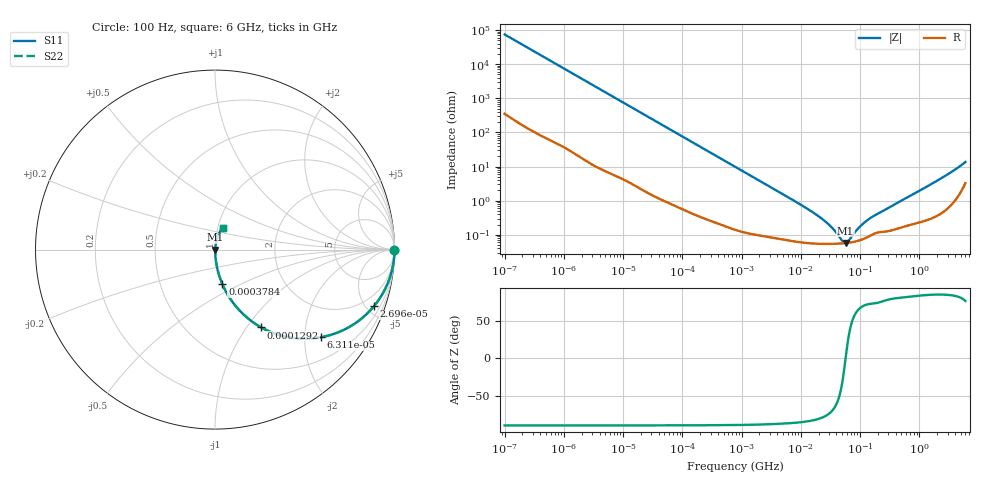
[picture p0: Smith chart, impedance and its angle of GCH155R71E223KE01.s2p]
!Murata Part Number: GCH155R71E223KE01
!These Parameters are Measured in Series Mode Connection
!Data Generated on Mar 13, 2026
!  o--ll--o
!Port1  Port2
!  o------o
!Operation Temp=25[degC], DC Bias Voltage=0[V]
!Freq. Start=100[Hz] Stop=6[GHz] 401[Steps]
# Hz S RI R 50
!Freq.(Hz) S11(Real) S11(Imag) S21(Real) S21(Imag) S12(Real) S12(Imag) S22(Real) S22(Imag)
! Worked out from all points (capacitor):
!   401 points, 100 Hz to 6 GHz, reference 50 ohm
!   read as one part in series: C = 21.5 nF near 109 Hz
!   lowest |Z| = 57.3 mohm at 56.99 MHz (marker M1)
!   series resonance near 57.05 MHz, so ESL is about 360 pH
!   S11 on the Smith chart (normalised r, x): 100 Hz: open; 26.96 kHz: 1.03, -5.59; 63.12 kHz: 1.02, -2.39; 129.2 kHz: 1.01, -1.17; 378.4 kHz: 1.00, -0.40; 6 GHz: 1.07, +0.26
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100  1 -0.00135  8.2e-06 0.00135  8.2e-06 0.00135  1 -0.00135
2008  0.9992 -0.0269  0.000848 0.0269  0.000848 0.0269  0.9992 -0.0269
8801  0.9858 -0.1156  0.0142 0.1156  0.0142 0.1156  0.9858 -0.1156
26957  0.8851 -0.316  0.1149 0.316  0.1149 0.316  0.8851 -0.316
40335  0.7762 -0.4137  0.2238 0.4137  0.2238 0.4137  0.7762 -0.4137
63115  0.5884 -0.4888  0.4116 0.4888  0.4116 0.4888  0.5884 -0.4888
90302  0.4131 -0.4888  0.5869 0.4888  0.5869 0.4888  0.4131 -0.4888
129199  0.2576 -0.4334  0.7424 0.4334  0.7424 0.4334  0.2576 -0.4334
211427  0.1165 -0.3163  0.8835 0.3163  0.8835 0.3163  0.1165 -0.3163
378399  0.0409 -0.1926  0.9591 0.1926  0.9591 0.1926  0.0409 -0.1926
774597  0.011 -0.0975  0.989 0.0975  0.989 0.0975  0.011 -0.0975
2481164  0.00186 -0.0309  0.9981 0.0309  0.9981 0.0309  0.00186 -0.0309
1.555665e7  0.000579 -0.00466  0.9994 0.00466  0.9994 0.00466  0.000579 -0.00466
2.911731e7  0.000545 -0.00199  0.9995 0.00199  0.9995 0.00199  0.000545 -0.00199
4.983056e7  0.000561 -0.000373  0.9994 0.000373  0.9994 0.000373  0.000561 -0.000373
5.699437e7  0.000573 -2.5e-06  0.9994 2.5e-06  0.9994 2.5e-06  0.000573 -2.5e-06
6.233367e7  0.000583 0.000244  0.9994 -0.000244  0.9994 -0.000244  0.000583 0.000244
8.918374e7  0.000657 0.00126  0.9993 -0.00126  0.9993 -0.00126  0.000657 0.00126
1.220122e8  0.000798 0.00225  0.9992 -0.00225  0.9992 -0.00225  0.000798 0.00225
3.124326e8  0.00134 0.00624  0.9987 -0.00624  0.9987 -0.00624  0.00134 0.00624
1.95892e9  0.0049 0.0372  0.9951 -0.0372  0.9951 -0.0372  0.0049 0.0372
6e9  0.0472 0.1217  0.9528 -0.1217  0.9528 -0.1217  0.0472 0.1217
